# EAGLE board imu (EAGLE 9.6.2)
REV: B
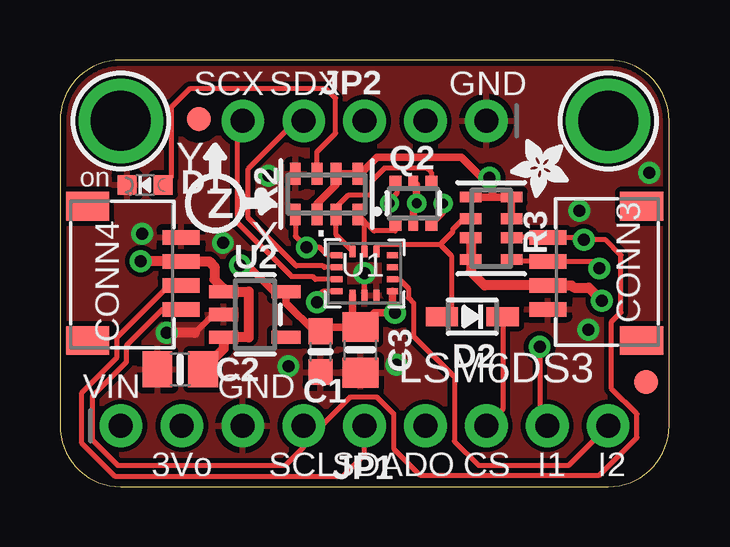
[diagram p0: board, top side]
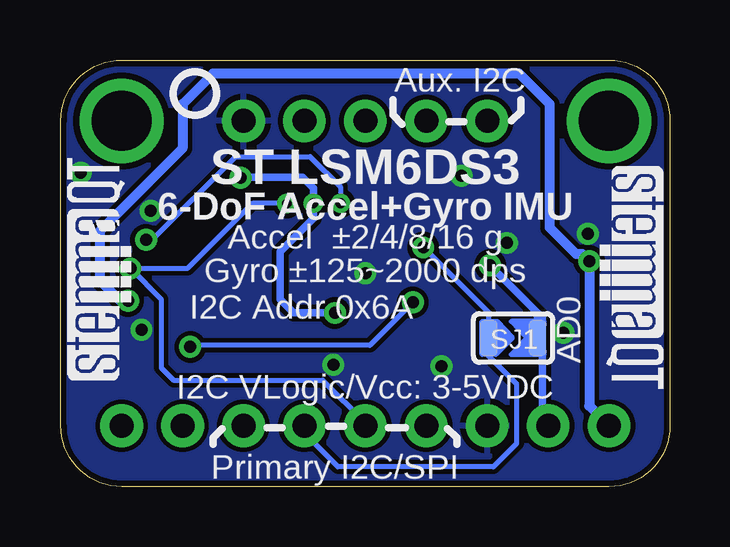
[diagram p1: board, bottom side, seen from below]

Size 25.4 x 17.78 mm. Coordinates in mm from the lower left corner, seen from the top.
Outline: 0,15.24 0,2.54 arc90 2.54,0 22.86,0 arc90 25.4,2.54 25.4,15.24 arc90 22.86,17.78 2.54,17.78 arc90 0,15.24
Copper layers (1*16): Top 0.035mm / dielectric 1.5mm / Bottom 0.035mm
Design rules "adafruit *": minimum track width 8mil, minimum drill 15.5mil, track to track 8mil, track to pad 8mil, pad to pad 8mil, via to via 8mil, smd to smd 8mil, copper to edge 10mil, drill to drill 8mil, minimum pad ring 10mil, minimum via ring 8mil, stop-mask expansion 2mil, vias tented up to drill 20mil, thermal gap 10mil
Net classes: 1 highpower: width 0.406 mm, drill 0.483 mm; 2 lowpower: width 0.305 mm, drill 0.483 mm

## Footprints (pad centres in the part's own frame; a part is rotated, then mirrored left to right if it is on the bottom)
0603-NO = smd 1.075 x 1: 1 -0.85,0; 2 0.85,0
0805-NO = smd 1.24 x 1.5: 1 -0.95,0; 2 0.95,0
JST_SH4 = smd 0.6 x 1.55: 1 -1.5,2.514; 2 -0.5,2.514; 3 0.5,2.514; 4 1.5,2.514 | smd 1.2 x 1.8: MT1 -2.8,-1.386; MT2 2.8,-1.386
CHIPLED_0603_NOOUTLINE = smd 0.8 x 0.8: A 0,-0.75; C 0,0.75
SOD-323 = smd 1.35 x 0.8: A 1.27,0; C -1.27,0
FIDUCIAL_1MM = smd 1 x 1: 1 0,0
1X09_ROUND_70 = drill 1 pad 1.778: 1 -10.16,0; 2 -7.62,0; 3 -5.08,0; 4 -2.54,0; 5 0,0; 6 2.54,0; 7 5.08,0; 8 7.62,0; 9 10.16,0
1X05_ROUND_70 = drill 1 pad 1.778: 1 -5.08,0; 2 -2.54,0; 3 0,0; 4 2.54,0; 5 5.08,0
SOT363 = smd 0.5 x 0.5: 1 -0.75,-0.9; 3 0.75,-0.9; 4 0.75,0.9; 6 -0.75,0.9 | smd 0.4 x 0.5: 2 0,-0.9; 5 0,0.9
RESPACK_4X0603 = smd 0.45 x 0.9: 1 -1.3,-0.85; 2 -0.4,-0.85; 3 0.4,-0.85; 4 1.3,-0.85; 5 1.3,0.85; 6 0.4,0.85; 7 -0.4,0.85; 8 -1.3,0.85
SOLDERJUMPER_ARROW_NOPASTE = smd 0.762 x 1.524: 1 -1.016,0; 2 1.016,0
LGA-14L = smd 0.475 x 0.25: 1 -1.163,0.75; 2 -1.163,0.25; 3 -1.163,-0.25; 4 -1.163,-0.75; 8 1.163,-0.75; 9 1.163,-0.25; 10 1.163,0.25; 11 1.163,0.75 | smd 0.25 x 0.475: 5 -0.5,-0.912; 6 0,-0.912; 7 0.5,-0.912; 12 0.5,0.912; 13 0,0.912; 14 -0.5,0.912
SOT23-5 = smd 0.55 x 1.2: 1 -0.95,-1.3; 2 0,-1.3; 3 0.95,-1.3; 4 0.95,1.3; 5 -0.95,1.3
MOUNTINGHOLE_2.5_PLATED = drill 2.5 pad 3.2: P$1 0,0

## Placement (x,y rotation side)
C1  0.1uF  [0603-NO]  10.86,5.63 270 top
C2  10uF  [0805-NO]  5.02,4.89 180 top
C3  10uF  [0805-NO]  12.52,5.7 270 top
CONN3  STEMMA_I2C_QT  [JST_SH4]  22.86,8.89 90 top
CONN4  STEMMA_I2C_QT  [JST_SH4]  2.54,8.89 270 top
D1  GREEN  [CHIPLED_0603_NOOUTLINE]  3.56,12.57 90 top
D2  1N4148  [SOD-323]  17.2,7.09 180 top
FID3  FIDUCIAL_1MM  [FIDUCIAL_1MM]  5.79,15.32 0 top
FID4  FIDUCIAL_1MM  [FIDUCIAL_1MM]  24.43,4.37 0 top
JP1  [1X09_ROUND_70]  12.7,2.54 0 top
JP2  [1X05_ROUND_70]  12.7,15.24 180 top
Q2  BSS138  [SOT363]  14.73,11.81 0 top
R2  10K  [RESPACK_4X0603]  11.11,12.19 180 top
R3  10K  [RESPACK_4X0603]  17.98,10.77 90 top
SJ1  [SOLDERJUMPER_ARROW_NOPASTE]  6.54,6.2 0 bottom
U1  LSM6DS3  [LGA-14L]  12.7,8.89 0 top
U2  AP2112K-3.3  [SOT23-5]  8.13,7.18 270 top
U$1  MOUNTINGHOLE2.5  [MOUNTINGHOLE_2.5_PLATED]  2.54,15.24 0 top
U$9  [ADAFRUIT_2.5MM]  21.21,14.48 180 top
U$17  MOUNTINGHOLE2.5  [MOUNTINGHOLE_2.5_PLATED]  22.86,15.24 0 top
U$25  [PCBFEAT-REV-040]  19.81,16.38 0 bottom
U$30  [STEMMAQT]  22.48,4.45 90 bottom
U$31  [STEMMAQT]  2.92,13.34 270 bottom

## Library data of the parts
C1-C3 CONN3 CONN4 D1 D2 JP1 JP2 Q2 R2 R3 U$9 U$25 = microbuilder
FID3 FID4 SJ1 = microbuilder; BOM: EXCLUDE
U1 = adafruit_sensor
U2 = adafruit_power
U$1 U$17 = adafruit_electromech; BOM: EXCLUDE
U$30 U$31 = silks

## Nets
3.3V [lowpower]: C1.1 C3.1 JP1.2 Q2.2 Q2.5 R2.1 R2.2 R2.6 R3.3 R3.4 R3.5 SJ1.2 U1.5 U1.8 U2.5
CS_3V: D2.A R3.6 U1.12
CS_5V: D2.C JP1.7
GND [highpower]: C1.2 C2.2 C3.2 CONN3.1 CONN4.1 D1.C JP1.3 JP2.1 R2.4 U1.6 U1.7 U2.2
INT1: JP1.8 U1.4
INT2: JP1.9 U1.9
N$1: D1.A R2.3
SCL: CONN3.4 CONN4.4 JP1.4 Q2.6 R3.2
SCL_3V: Q2.1 R2.8 U1.13
SCX: JP2.5 U1.3
SDA: CONN3.3 CONN4.3 JP1.5 Q2.3 R3.1
SDA_3V: Q2.4 R2.7 U1.14
SDO: JP1.6 R2.5 SJ1.1 U1.1
SDX: JP2.4 U1.2
VCC [highpower]: C2.1 CONN3.2 CONN4.2 JP1.1 R3.7 R3.8 U2.1 U2.3

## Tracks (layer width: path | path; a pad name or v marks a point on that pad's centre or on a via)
3.3V  (via drill 0.4, 0.5)
  Top 0.305: U1.5 12.2,6.97 C3.1 | Q2.5 14.87,12.57 v14.87,11.81 14.73,11.68 Q2.2 | v7.51,9.23 7.82,9.23 8.93,8.13 U2.5 9.43,7.65 10.61,6.48 C1.1 11.04,6.65 C3.1 | R2.6 10.71,11.79 11.51,12.59 R2.2 R2.1 12.54,13.04 13.23,13.73 16.73,13.73 17.59,12.87 v17.91,12.87 18.03,12.75 18.03,12.07 | R3.3 R3.4 | R3.4 | R3.5 18.03,12.07 | 18.03,12.07 R3.4 | C3.1 13.11,7.24 13.78,7.24 | 13.78,7.24 v13.97,7.24 | U1.8 13.86,7.32 13.78,7.24
  Bottom 0.305: JP1.2 5.32,2.78 5.32,7.04 v7.51,9.23 5.52,7.25 SJ1.2 | v13.97,7.24 15.68,7.24 16.26,7.81 16.26,9.79 14.87,11.18 v14.87,11.81 14.87,12.45 15.31,12.89 17.89,12.89 v17.91,12.87
CS_3V
  Top 0.203: U1.12 13.2,10.03 13.27,10.1 15.85,10.1 | 15.85,10.1 16.32,9.63 16.32,7.48 D2.A | 15.85,10.1 15.86,10.1 16.38,10.62 16.38,10.72 16.83,11.17 R3.6
CS_5V
  Top 0.203: JP1.7 18.47,3.23 D2.C
GND  (via drill 0.5)
  Top 0.203: U1.6 v12.7,8.89
  Top 0.254: 6.75,7.1 6.31,7.1 5.63,6.41
  Top 0.406: U2.2 6.75,7.1 | 5.63,6.41 v4.45,6.41
  other vias: 3.43,10.54 21.65,11.49 22.03,6.54 24.57,13.08 6.79,10.16 8.7,12.95 14.03,5.08 9.53,5.02
  pour Top: 0,17.78 25.4,17.78 25.4,0 0,0
  pour Bottom: 0,17.78 25.4,17.78 25.4,0 0,0
INT1  (via drill 0.5)
  Top 0.203: U1.4 10.97,8.14 10.72,7.89 v10.72,7.68 | v20,5.83 20,2.86 JP1.8
  Bottom 0.203: v10.72,7.68 12.51,5.89 19.94,5.89 v20,5.83
INT2
  Top 0.203: JP1.9 21.21,0.89 17.46,0.89 16.45,1.91 16.45,4.57 14.74,6.27 14.74,7.65 14.52,7.87 14.52,8.27 14.16,8.64 U1.9
N$1
  Top 0.203: D1.A 4.64,12.9 4.64,15.81 5.4,16.57 11.11,16.57 11.49,16.19 11.49,14.73 10.71,13.95 R2.3
SCL  (via drill 0.4, 0.5)
  Top 0.203: Q2.6 14.05,12.65 14.05,12.22 13.74,11.91 v13.74,11.81 | CONN4.4 4.28,7.39 2.77,5.88 2.77,5.2 1.35,3.78 1.35,1.96 2.42,0.89 9.4,0.89 10.16,1.65 JP1.4 10.92,2.54 12.12,3.75 13.21,3.75 13.91,3.05 13.91,1.59 15.01,0.48 22.49,0.48 24.05,2.05 24.05,3.03 23,4.09 23,6.87 23.39,7.26 23.39,9.65 22.76,10.29 v21.84,10.29 21.74,10.39 CONN3.4 18.85,10.39 R3.2
  Bottom 0.203: v21.84,10.29 21.59,10.29 18.12,13.76 15.01,13.76 13.74,12.49 v13.74,11.81
SCL_3V
  Top 0.203: 13.98,10.66 13.1,10.66 R2.8 12.7,11.05 U1.13 | Q2.1 13.98,10.66 | 13.98,10.66
SCX
  Top 0.203: U1.3 10.65,8.64 10.52,8.77 9.65,8.77 7.39,11.02 7.39,14.93 7.62,15.16 JP2.5
SDA  (via drill 0.4, 0.5)
  Top 0.203: R3.1 18.91,9.39 CONN3.3 22.49,9.39 v22.49,9.09 | Q2.3 15.97,11.4 v15.97,11.8 | CONN4.3 4.55,8.39 2.36,6.2 2.36,5.36 0.89,3.89 0.89,1.84 2.29,0.45 11.81,0.45 12.7,1.33 JP1.5
  Bottom 0.203: v15.97,11.8 17.41,11.8 20.12,9.09 v22.49,9.09 21.21,7.81 21.21,4.95 20.7,4.45 14.48,4.45 12.7,2.67 JP1.5
SDA_3V
  Top 0.203: Q2.4 15.48,13.09 15.3,13.27 13.53,13.27 13.01,12.75 13.01,12.16 12.03,12.16 11.51,11.64 R2.7 11.51,10.49 U1.14
SDO  (via drill 0.5)
  Top 0.203: U1.1 11.16,9.64 10.83,9.97 v10.29,9.97 9.81,10.44 R2.5
  Bottom 0.203: JP1.6 15.24,2.22 13.84,0.83 7.37,0.83 6.39,1.8 6.39,4.27 7.56,5.44 SJ1.1 7.56,7.24 v10.29,9.97
SDX
  Top 0.203: U1.2 11.03,9.14 10.97,9.2 9.85,9.2 7.85,11.2 7.85,13.24 9.85,15.24 JP2.4
VCC  (via drill 0.5)
  Top 0.406: R3.7 R3.8 17.13,8.96 17.7,8.39 CONN3.2 21.33,8.39 21.43,8.29 22.05,8.29 v22.59,7.75 | C2.1 6.83,5.75 U2.3 7.87,6.23 7.87,8.13 U2.1 6.83,8.25 6.45,8.63 6.45,9.17 6.23,9.39 CONN4.2 v3.37,9.39 v3.37,9.4
  Bottom 0.406: JP1.1 3.37,3.37 v3.37,9.4 3.66,9.69 3.91,9.69 5.02,10.8 5.02,15.94 6.29,17.21 19.05,17.21 20.32,15.94 20.32,14.1 23.75,10.67 23.75,8.57 22.92,7.75 v22.59,7.75

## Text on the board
tPlace: SCX | SDX | GND | on | Y | Z | X | LSM6DS3 | VIN | GND | 3Vo | SCL | SDA | DO | CS | I1 | I2
bPlace: Aux. I2C | ST LSM6DS3 | 6-DoF Accel+Gyro IMU | Accel ±2/4/8/16 g | Gyro ±125~2000 dps | AD0 | I2C Addr 0x6A | I2C VLogic/Vcc: 3-5VDC | Primary I2C/SPI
